[IBIS Ver]   3.2
[File Name]   sprm149a.ibs
[File Rev]   0.2
[Date]   July 2, 2004
[Disclaimer]   Please be aware that in the absence of a written agreement
|   Texas Instruments(TI) assumes no liability for:
|   (1) The accuracy of the IBIS models provided to your company
|   (2) The proper functioning of these Models in your design
|   or for any resulting applications
|   (3) Infringement of patents, copyrights or intellectual
|   property rights resulting from your use of these
|   models.
|   TI provides IBIS Models as a service to our customers and
|   therefore reserves the right to limit distribution of the
|   Models.
[Copyright]   Property of Texas Instruments Incorporated.
|   Unauthorized reproduction and/or distribution is strictly.
|   prohibited.
|   This product is protected under copyright law and trade
|   secret law as an unpublished work.
|   Created 2003,(C) Copyright 1999-2004,
|   Texas Instruments Incorporated., All Rights Reserved.
|   These commodities are under the U.S. Government
|   distribution license control. As such,they are not to be
|   re-exported without the prior approval of the U.S.
|   Department of Commerce.
[Notes]
|   File Rev 0.1   Initial revision
|   File Rev 0.2   Renamed EMIF address pins from AEA[21:2] to
|   AEA[22:3] for compatibility with EMIF
|   documentation for EMIFA.  Note that the
|   C6410 is still a 32-bit interface, this is
|   just a pin name change.
|****** ****   ***** *****   ******  Package Models  **************************
[Component]   C6410_GTS
[Manufacturer]  Texas Instruments
[Package]
|Variable   Typ   Min   Max
R_pkg   3.344e-01   3.561e-03   6.407e-01
L_pkg   3.999e-09   2.752e-10   8.538e-09
C_pkg   5.967e-13   2.696e-13   2.294e-12
[Pin]   signal_name   model_name   R_pin   L_pin   C_pin
A11   CLKINSEL   IT33THYPU   3.61E-01   6.05E-09   3.93E-13
A12   CLKIN   IT33THYPD   3.13E-01   3.83E-09   6.54E-13
A13   CLKMODE1   IT33THYPD   3.21E-01   3.59E-09   7.02E-13
A15   AED06   BT3315DTPU   3.56E-01   3.63E-09   7.44E-13
A16   AED03   BT3315DTPU   3.24E-01   3.91E-09   7.72E-13
A18   AED15   BT3315DTPU   3.62E-01   4.54E-09   7.53E-13
A19   AED11   BT3315DTPU   3.68E-01   4.75E-09   7.77E-13
A2   CLKOUT4_GP0_01   BT3315DTHYPU   5.06E-01   7.69E-09   6.52E-13
A21   AED08   BT3315DTPU   4.14E-01   4.79E-09   8.38E-13
A22   ABE1Z   BT3315DTPU   5.02E-01   5.24E-09   9.21E-13
A4   GP0_04_EXT_INT4   BT3325CTHYPU   3.02E-01   4.30E-09   7.88E-13
AA1   TOUT1_LENDIAN   BT3325CTPU   4.14E-01   8.54E-09   5.63E-13
AA11   ACLKR1_2_HCSZ   IT33THYPU   2.76E-01   5.67E-09   3.30E-13
AA12   GP0_14_HD14   BT3325CTHYPU   2.88E-01   5.58E-09   3.29E-13
AA13   HD06   BT3325CTHYPU   4.00E-01   5.19E-09   3.49E-13
AA14   HD04   BT3325CTHYPU   4.53E-01   3.79E-09   4.93E-13
AA15   GP0_10_HD10   BT3325CTHYPU   4.87E-01   4.27E-09   4.97E-13
AA16   HD02   BT3325CTHYPU   4.52E-01   4.17E-09   5.36E-13
AA18   SCL1   BQ0001THY   3.28E-01   4.55E-09   7.45E-13
AA19   SDA1   BQ0001THY   2.62E-01   4.27E-09   9.54E-13
AA2   TOUT0   BT3325CTPD   5.39E-01   4.33E-09   6.84E-13
AA21   AED25   BT3315DTPU   3.94E-01   4.57E-09   8.79E-13
AA22   AED27   BT3315DTPU   6.38E-01   4.81E-09   7.99E-13
AA4   ACLKX1_HD24   BT3325CTHYPU   4.79E-01   3.75E-09   7.25E-13
AA5   AFSR1_3_HRWZ   IT33THYPU   2.45E-01   4.06E-09   6.53E-13
AA6   AXR1_03_HD19   BT3325CTHYPU   2.32E-01   3.90E-09   6.04E-13
AA7   AXR1_01_HD17   BT3325CTHYPU   2.21E-01   3.91E-09   5.21E-13
AA8   HINTZ   BT3325CTHYPU   5.04E-01   3.49E-09   5.87E-13
AA9   ACLKR1_HD25   BT3325CTHYPU   2.05E-01   3.75E-09   5.23E-13
AB1   TINP1   IT33THYPD   6.05E-01   4.42E-09   1.05E-12
AB11   ACLKR1_3_HDS1Z   IT33THYPU   4.06E-01   6.57E-09   3.62E-13
AB12   HDS2Z   IT33THYPU   3.07E-01   6.64E-09   3.63E-13
AB13   GP0_13_HD13   BT3325CTHYPU   5.02E-01   6.17E-09   3.73E-13
AB14   GP0_11_HD11   BT3325CTHYPU   4.14E-01   4.31E-09   5.70E-13
AB15   HD03   BT3325CTHYPU   5.42E-01   4.37E-09   6.05E-13
AB16   GP0_08_HD08   BT3325CTHYPU   3.82E-01   4.61E-09   5.74E-13
AB18   SCL0   BQ0001THY   3.47E-01   4.07E-09   8.47E-13
AB19   SDA0   BQ0001THY   5.57E-01   4.91E-09   7.37E-13
AB2   TINP0   IT33THYPD   4.01E-01   4.79E-09   7.85E-13
AB21   ABE3Z   BT3315DTPU   6.24E-01   5.14E-09   8.91E-13
AB22   AED24   BT3315DTPU   4.19E-01   5.28E-09   7.69E-13
AB4   AHCLKR1_HD26   BT3325CTHYPU   4.51E-01   4.57E-09   7.58E-13
AB5   AFSX1_HD22   BT3325CTHYPU   4.27E-01   4.35E-09   7.19E-13
AB6   AXR1_00_HD16   BT3325CTHYPU   2.75E-01   4.08E-09   6.58E-13
AB7   AXR1_02_HD18   BT3325CTHYPU   4.57E-01   4.18E-09   6.49E-13
AB8   AXR1_04_HD20   BT3325CTHYPU   5.20E-01   3.94E-09   7.77E-13
AB9   AFSR1_HD23   BT3325CTHYPU   2.45E-01   3.81E-09   7.72E-13
B10   CLKMODE2   IT33THYPD   2.65E-01   2.96E-09   5.50E-13
B13   GP0_03   BT3325CTHYPD   2.83E-01   3.10E-09   5.59E-13
B15   AED05   BT3315DTPU   2.89E-01   3.59E-09   6.21E-13
B16   AED01   BT3315DTPU   2.94E-01   3.69E-09   6.39E-13
B18   AED13   BT3315DTPU   3.18E-01   7.53E-09   3.93E-13
B19   AED09   BT3315DTPU   3.25E-01   6.68E-09   4.47E-13
B21   AEA12   BT3315DTPD   4.64E-01   4.55E-09   7.68E-13
B22   AEA11   BT3315DTPD   4.18E-01   5.18E-09   7.83E-13
B3   CLKOUT6_GP0_02   BT3315DTHYPU   2.78E-01   6.68E-09   5.03E-13
B4   GP0_05_EXT_INT5   BT3325CTHYPU   2.72E-01   4.10E-09   6.77E-13
B7   OSC_DIS   IT33THYPU   2.89E-01   3.55E-09   6.89E-13
B9   NMI   IT33THYPD   2.56E-01   2.93E-09   5.79E-13
C11   CLKMODE3   IT33THYPD   1.88E-01   2.63E-09   6.50E-13
C13   CLKMODE0   IT33THYPD   3.81E-01   4.26E-09   3.43E-13
C15   AED04   BT3315DTPU   2.44E-01   4.68E-09   3.61E-13
C16   AED02   BT3315DTPU   2.51E-01   4.93E-09   3.63E-13
C17   AED00   BT3315DTPU   2.65E-01   3.29E-09   5.59E-13
C18   AED12   BT3315DTPU   2.84E-01   6.45E-09   3.71E-13
C19   AED10   BT3315DTPU   5.15E-01   6.35E-09   4.24E-13
C2   CLKR0   BT3325CTHYPD   2.89E-01   6.91E-09   5.95E-13
C20   AAWEZ_ASDWEZ_ASWEZ   BT3315DTPU   3.55E-01   3.93E-09   7.82E-13
C4   GP0_06_EXT_INT6   BT3325CTHYPU   2.37E-01   5.51E-09   5.59E-13
D1   FSR0   BT3325CTHYPD   3.18E-01   4.19E-09   7.31E-13
D13   GP0_00   BT3325CTHYPD   1.74E-01   3.43E-09   3.69E-13
D15   AED07   BT3315DTPU   2.80E-01   4.62E-09   2.99E-13
D16   ABE0Z   BT3315DTPU   2.63E-01   2.47E-09   4.97E-13
D17   AED14   BT3315DTPU   2.92E-01   1.25E-09   4.68E-13
D2   DR0   IT33THYPD   2.77E-01   3.98E-09   6.83E-13
D20   AAREZ_ASDCASZ_ASADSZ   BT3315DTPU   2.71E-01   6.08E-09   3.91E-13
D21   AEA10   BT3315DTPD   3.52E-01   3.89E-09   7.73E-13
D22   AEA09   BT3315DTPD   3.81E-01   4.23E-09   8.24E-13
D3   CLKS0   IT33THYPD   2.64E-01   6.85E-09   3.54E-13
E2   DX0   BT3325CTHYPD   4.61E-01   3.73E-09   7.00E-13
E20   AAOEZ_ASDRASZ_ASOEZ   BT3315DTPU   5.76E-01   6.14E-09   3.83E-13
E21   AEA08   BT3315DTPD   3.44E-01   3.82E-09   6.59E-13
E22   AEA07   BT3315DTPD   3.76E-01   4.51E-09   7.09E-13
E3   CLKX0   BT3325CTHYPD   3.93E-01   3.30E-09   6.39E-13
E4   FSX0   BT3325CTHYPD   1.96E-01   5.58E-09   3.25E-13
F1   DR1   IT33THYPD   2.71E-01   4.25E-09   7.48E-13
F20   ACE0Z   BT3315DTPU   4.69E-01   3.33E-09   5.55E-13
F21   AEA06   BT3315DTPD   3.24E-01   3.67E-09   6.48E-13
F22   AECLKOUT1   BT3315DTPD   3.52E-01   4.05E-09   6.93E-13
G1   CLKS1   IT33THYPD   3.22E-01   3.93E-09   7.63E-13
G2   FSR1   BT3325CTHYPD   2.31E-01   3.42E-09   5.82E-13
G20   AEA14   BT3315DTPD   2.79E-01   2.94E-09   5.83E-13
G3   CLKR1   BT3325CTHYPD   2.03E-01   3.13E-09   5.22E-13
H1   CLKX1   BT3325CTHYPD   3.17E-01   3.79E-09   7.73E-13
H19   ACE3Z   BT3315DTPU   2.85E-01   2.24E-09   4.61E-13
H2   DX1   BT3325CTHYPD   2.78E-01   3.50E-09   5.60E-13
H20   AEA15   BT3315DTPD   2.89E-01   2.92E-09   5.72E-13
H21   AEA17   BT3315DTPD   4.49E-01   3.32E-09   6.93E-13
H22   AEA18   BT3315DTPD   5.57E-01   3.98E-09   7.72E-13
H3   FSX1   BT3325CTHYPD   2.44E-01   2.82E-09   5.02E-13
J19   AEA04   BT3315DTPD   3.42E-01   2.12E-09   5.03E-13
J20   AEA16   BT3315DTPD   2.69E-01   2.74E-09   5.50E-13
J21   AHOLDAZ   BT3315DTPU   3.02E-01   3.32E-09   5.72E-13
J22   AHOLDZ   IT33THYPU   3.45E-01   3.90E-09   6.54E-13
J4   AMUTEIN0   IT33THYPD   1.64E-01   4.03E-09   2.81E-13
K1   ACLKR0   BT3325CTHYPD   2.71E-01   3.81E-09   5.70E-13
K2   AFSR0   BT3325CTHYPD   3.77E-01   2.91E-09   5.27E-13
K20   AEA13   BT3315DTPD   4.23E-01   2.51E-09   5.71E-13
K21   ASDCKE   BT3315DTPU   6.02E-01   3.08E-09   5.70E-13
K22   AECLKIN   IT33THYPD   3.92E-01   3.27E-09   6.26E-13
K3   AXR0_1   BT3325CTHYPD   1.91E-01   4.94E-09   3.03E-13
K4   AMUTE0   BT3325CTHYPD   1.53E-01   3.87E-09   2.70E-13
L1   AHCLKR0   BT3325CTHYPD   2.75E-01   3.55E-09   7.10E-13
L2   AXR0_0   BT3325CTHYPD   2.55E-01   2.96E-09   5.53E-13
L20   AEA03   BT3315DTPD   2.54E-01   2.66E-09   5.93E-13
L21   AARDY   IT33THYPU   2.83E-01   3.02E-09   5.28E-13
L3   AXR0_2   BT3325CTHYPD   3.65E-01   2.41E-09   5.90E-13
M1   ACLKX0   BT3325CTHYPD   2.91E-01   3.80E-09   6.06E-13
M2   AFSX0   BT3325CTHYPD   5.09E-01   3.25E-09   6.09E-13
M20   AEA05   BT3315DTPD   2.29E-01   4.27E-09   3.41E-13
M21   AEA22   BT3315DTPD   3.04E-01   3.13E-09   5.70E-13
M3   AXR0_3   BT3325CTHYPD   2.77E-01   4.65E-09   3.45E-13
N1   AHCLKX0   BT3325CTHYPD   6.41E-01   3.44E-09   6.68E-13
N20   ACE2Z   BT3315DTPU   2.75E-01   2.50E-09   5.63E-13
N21   AEA21   BT3315DTPD   3.11E-01   3.21E-09   5.26E-13
N22   AEA19   BT3315DTPD   3.30E-01   3.69E-09   6.91E-13
N3   AXR0_4   BT3325CTHYPD   2.81E-01   4.35E-09   3.43E-13
P19   ASOE3Z   BT3315DTPU   1.62E-01   2.40E-09   4.81E-13
P2   EMU5   BT3315DTHYPU   5.20E-01   3.15E-09   6.92E-13
P20   AED23   BT3315DTPU   2.64E-01   2.96E-09   4.91E-13
P21   ABE2Z   BT3315DTPU   3.28E-01   3.14E-09   6.03E-13
P22   AEA20   BT3315DTPD   3.37E-01   3.64E-09   7.94E-13
P3   AXR0_5   BT3325CTHYPD   2.78E-01   2.91E-09   5.36E-13
R1   EMU0   BT3315DTHYPU   4.33E-01   3.70E-09   7.41E-13
R19   ABUSREQ   BT3315DTPU   2.18E-01   4.46E-09   2.93E-13
R2   EMU2   BT3315DTHYPU   4.58E-01   3.44E-09   7.01E-13
R20   ACE1Z   BT3315DTPU   2.42E-01   2.83E-09   5.35E-13
R21   AED21   BT3315DTPU   3.37E-01   3.30E-09   6.02E-13
R22   AED22   BT3315DTPU   3.44E-01   3.92E-09   6.78E-13
R3   EMU4   BT3315DTHYPU   2.94E-01   3.02E-09   5.42E-13
R4   EMU6   BT3315DTHYPU   2.91E-01   4.13E-09   3.54E-13
T1   TDI   IT33THYPU   5.60E-01   3.85E-09   7.65E-13
T19   APDTDZ   BT3315DTPU   3.77E-01   1.72E-09   4.57E-13
T2   TCK   IT33THYPU   3.43E-01   3.28E-09   7.50E-13
T20   AED18   BT3315DTPU   2.58E-01   3.02E-09   5.43E-13
T3   EMU1   BT3315DTHYPU   2.47E-01   3.13E-09   5.15E-13
T4   TDO   BT3325CTPU   2.87E-01   1.83E-09   3.78E-13
U1   TRSTZ   IT33THYPD   4.83E-01   4.14E-09   6.77E-13
U2   EMU3   BT3315DTHYPU   2.23E-01   6.78E-09   3.60E-13
U20   AED16   BT3315DTPU   2.79E-01   3.10E-09   6.08E-13
U21   AED20   BT3315DTPU   3.13E-01   3.75E-09   6.44E-13
U22   AECLKOUT2   BT3315DTPD   3.35E-01   3.97E-09   7.00E-13
U3   TMS   IT33THYPU   2.47E-01   3.27E-09   5.33E-13
V1   EMU8   BT3315DTHYPU   3.75E-01   4.30E-09   8.35E-13
V2   EMU7   BT3315DTHYPU   3.67E-01   3.69E-09   7.04E-13
V20   AED29   BT3315DTPU   3.05E-01   3.26E-09   6.40E-13
V21   AED19   BT3315DTPU   3.26E-01   3.81E-09   7.40E-13
V22   AED17   BT3315DTPU   3.43E-01   4.41E-09   7.47E-13
V3   EMU9   BT3315DTHYPU   3.22E-01   6.21E-09   3.58E-13
W10   AMUTE1_HD28   BT3325CTHYPU   3.28E-01   3.88E-09   2.78E-13
W11   AMUTEIN1_HD29   BT3325CTHYPU   1.23E-01   3.83E-09   2.70E-13
W12   HD07   BT3325CTHYPU   1.46E-01   1.06E-09   4.53E-13
W15   HD00   BT3325CTHYPU   5.08E-01   2.76E-09   4.10E-13
W2   EMU11   BT3315DTHYPU   3.03E-01   7.25E-09   3.89E-13
W20   AED28   BT3315DTPU   2.37E-01   5.67E-09   4.09E-13
W21   AED31   BT3315DTPU   3.40E-01   3.81E-09   7.02E-13
W22   AED30   BT3315DTPU   3.49E-01   4.29E-09   7.81E-13
W3   EMU10   BT3315DTHYPU   5.59E-01   6.46E-09   3.69E-13
W7   HCNTL1   IT33THYPU   4.47E-01   2.83E-09   4.76E-13
Y1   GP0_07_EXT_INT7   BT3325CTHYPU   4.73E-01   7.26E-09   5.87E-13
Y10   HRDYZ   BT3325CTHYPU   2.42E-01   4.29E-09   3.82E-13
Y11   HD30   BT3325CTHYPU   2.42E-01   4.77E-09   3.05E-13
Y12   GP0_15_HD15   BT3325CTHYPU   2.51E-01   4.73E-09   3.02E-13
Y13   HD05   BT3325CTHYPU   1.50E-01   3.73E-09   3.32E-13
Y14   GP0_12_HD12   BT3325CTHYPU   3.70E-01   3.36E-09   5.23E-13
Y15   HD01   BT3325CTHYPU   4.45E-01   3.48E-09   4.25E-13
Y16   GP0_09_HD09   BT3325CTHYPU   3.14E-01   3.67E-09   5.50E-13
Y20   AED26   BT3315DTPU   3.12E-01   3.85E-09   8.38E-13
Y4   AHCLKX1_HD27   BT3325CTHYPU   3.29E-01   5.76E-09   3.96E-13
Y5   ACLKR1_1_HASZ   IT33THYPU   4.99E-01   3.65E-09   8.21E-13
Y6   AFSR1_1_HCNTL0   IT33THYPU   2.74E-01   3.38E-09   5.83E-13
Y7   AFSR1_2_HHWIL   IT33THYPU   3.25E-01   2.82E-09   5.25E-13
Y8   HD31   BT3325CTHYPU   2.56E-01   2.79E-09   6.61E-13
Y9   AXR1_05_HD21   BT3325CTHYPU   4.94E-01   4.46E-09   3.58E-13
| Models and submodels in the file (10): BQ0001THY (I/O_open_sink), BT3315DTHYPU (I/O), BT3315DTPD (I/O), BT3315DTPU (I/O), BT3325CTHYPD (I/O), BT3325CTHYPU (I/O), BT3325CTPD (I/O), BT3325CTPU (I/O), IT33THYPD (Input), IT33THYPU (Input)
